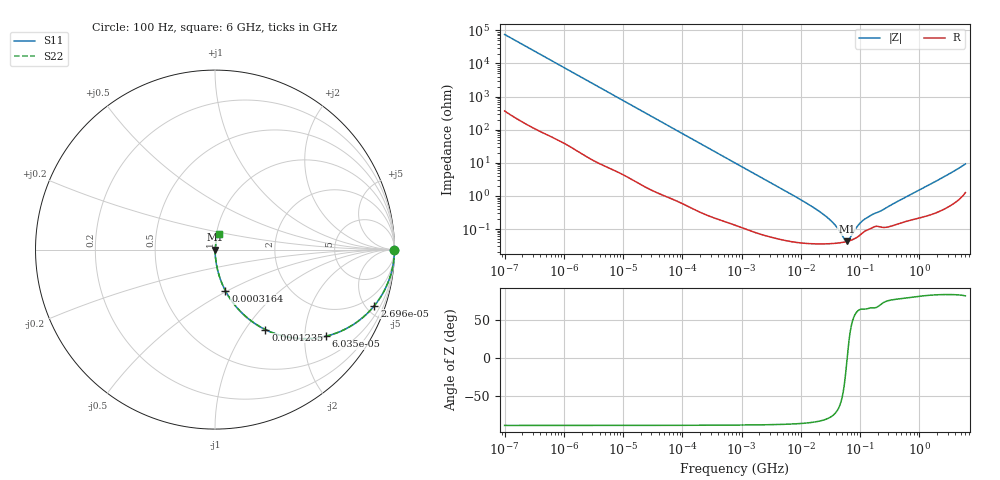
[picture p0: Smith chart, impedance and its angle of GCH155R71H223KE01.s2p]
!Murata Part Number: GCH155R71H223KE01
!These Parameters are Measured in Series Mode Connection
!Data Generated on Mar 13, 2026
!  o--ll--o
!Port1  Port2
!  o------o
!Operation Temp=25[degC], DC Bias Voltage=0[V]
!Freq. Start=100[Hz] Stop=6[GHz] 401[Steps]
# Hz S RI R 50
!Freq.(Hz) S11(Real) S11(Imag) S21(Real) S21(Imag) S12(Real) S12(Imag) S22(Real) S22(Imag)
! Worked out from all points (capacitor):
!   401 points, 100 Hz to 6 GHz, reference 50 ohm
!   read as one part in series: C = 21.2 nF near 109 Hz
!   lowest |Z| = 42.4 mohm at 59.6 MHz (marker M1)
!   series resonance near 60.61 MHz, so ESL is about 330 pH
!   S11 on the Smith chart (normalised r, x): 100 Hz: open; 26.96 kHz: 1.03, -5.67; 60.35 kHz: 1.02, -2.54; 123.5 kHz: 1.01, -1.25; 316.4 kHz: 1.00, -0.49; 6 GHz: 1.03, +0.18
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100  1 -0.00133  8.3e-06 0.00133  8.3e-06 0.00133  1 -0.00133
2008  0.9992 -0.0265  0.000833 0.0265  0.000833 0.0265  0.9992 -0.0265
8801  0.9862 -0.1139  0.0138 0.1139  0.0138 0.1139  0.9862 -0.1139
26957  0.888 -0.3125  0.112 0.3125  0.112 0.3125  0.888 -0.3125
40335  0.7812 -0.4103  0.2188 0.4103  0.2188 0.4103  0.7812 -0.4103
60352  0.6166 -0.4828  0.3834 0.4828  0.3834 0.4828  0.6166 -0.4828
86348  0.4421 -0.4929  0.5579 0.4929  0.5579 0.4929  0.4421 -0.4929
123542  0.281 -0.4456  0.719 0.4456  0.719 0.4456  0.281 -0.4456
193316  0.1393 -0.3421  0.8607 0.3421  0.8607 0.3421  0.1393 -0.3421
316350  0.0582 -0.2294  0.9418 0.2294  0.9418 0.2294  0.0582 -0.2294
774597  0.0112 -0.099  0.9888 0.099  0.9888 0.099  0.0112 -0.099
2481164  0.00163 -0.0314  0.9984 0.0314  0.9984 0.0314  0.00163 -0.0314
1.555665e7  0.000384 -0.00475  0.9996 0.00475  0.9996 0.00475  0.000384 -0.00475
3.330331e7  0.000368 -0.00166  0.9996 0.00166  0.9996 0.00166  0.000368 -0.00166
4.165952e7  0.000379 -0.001  0.9996 0.001  0.9996 0.001  0.000379 -0.001
5.449875e7  0.000407 -0.000279  0.9996 0.000279  0.9996 0.000279  0.000407 -0.000279
5.960426e7  0.000422 -4.33e-05  0.9996 4.33e-05  0.9996 4.33e-05  0.000422 -4.33e-05
6.518806e7  0.000441 0.000192  0.9996 -0.000192  0.9996 -0.000192  0.000441 0.000192
8.918374e7  0.000569 0.00104  0.9994 -0.00104  0.9994 -0.00104  0.000569 0.00104
1.115611e8  0.000782 0.00164  0.9992 -0.00164  0.9992 -0.00164  0.000782 0.00164
3.124326e8  0.00121 0.00485  0.9988 -0.00485  0.9988 -0.00485  0.00121 0.00485
6e9  0.0206 0.0892  0.9794 -0.0892  0.9794 -0.0892  0.0206 0.0892
